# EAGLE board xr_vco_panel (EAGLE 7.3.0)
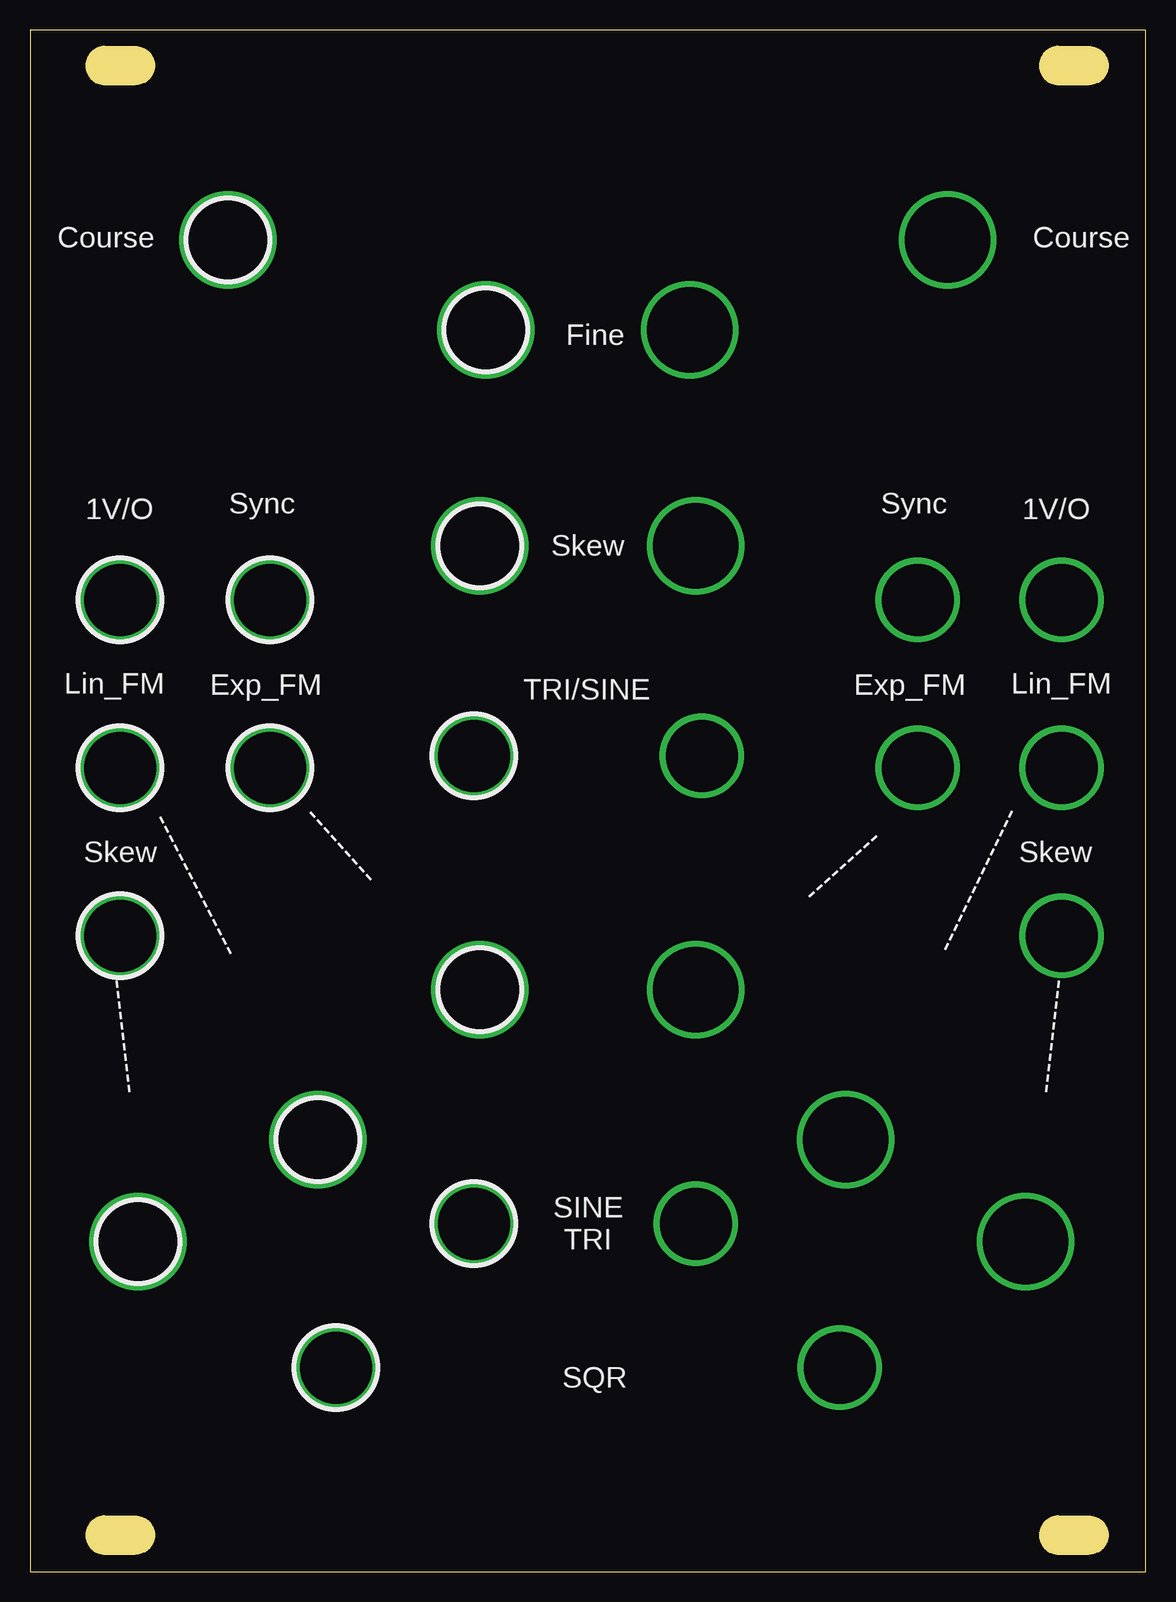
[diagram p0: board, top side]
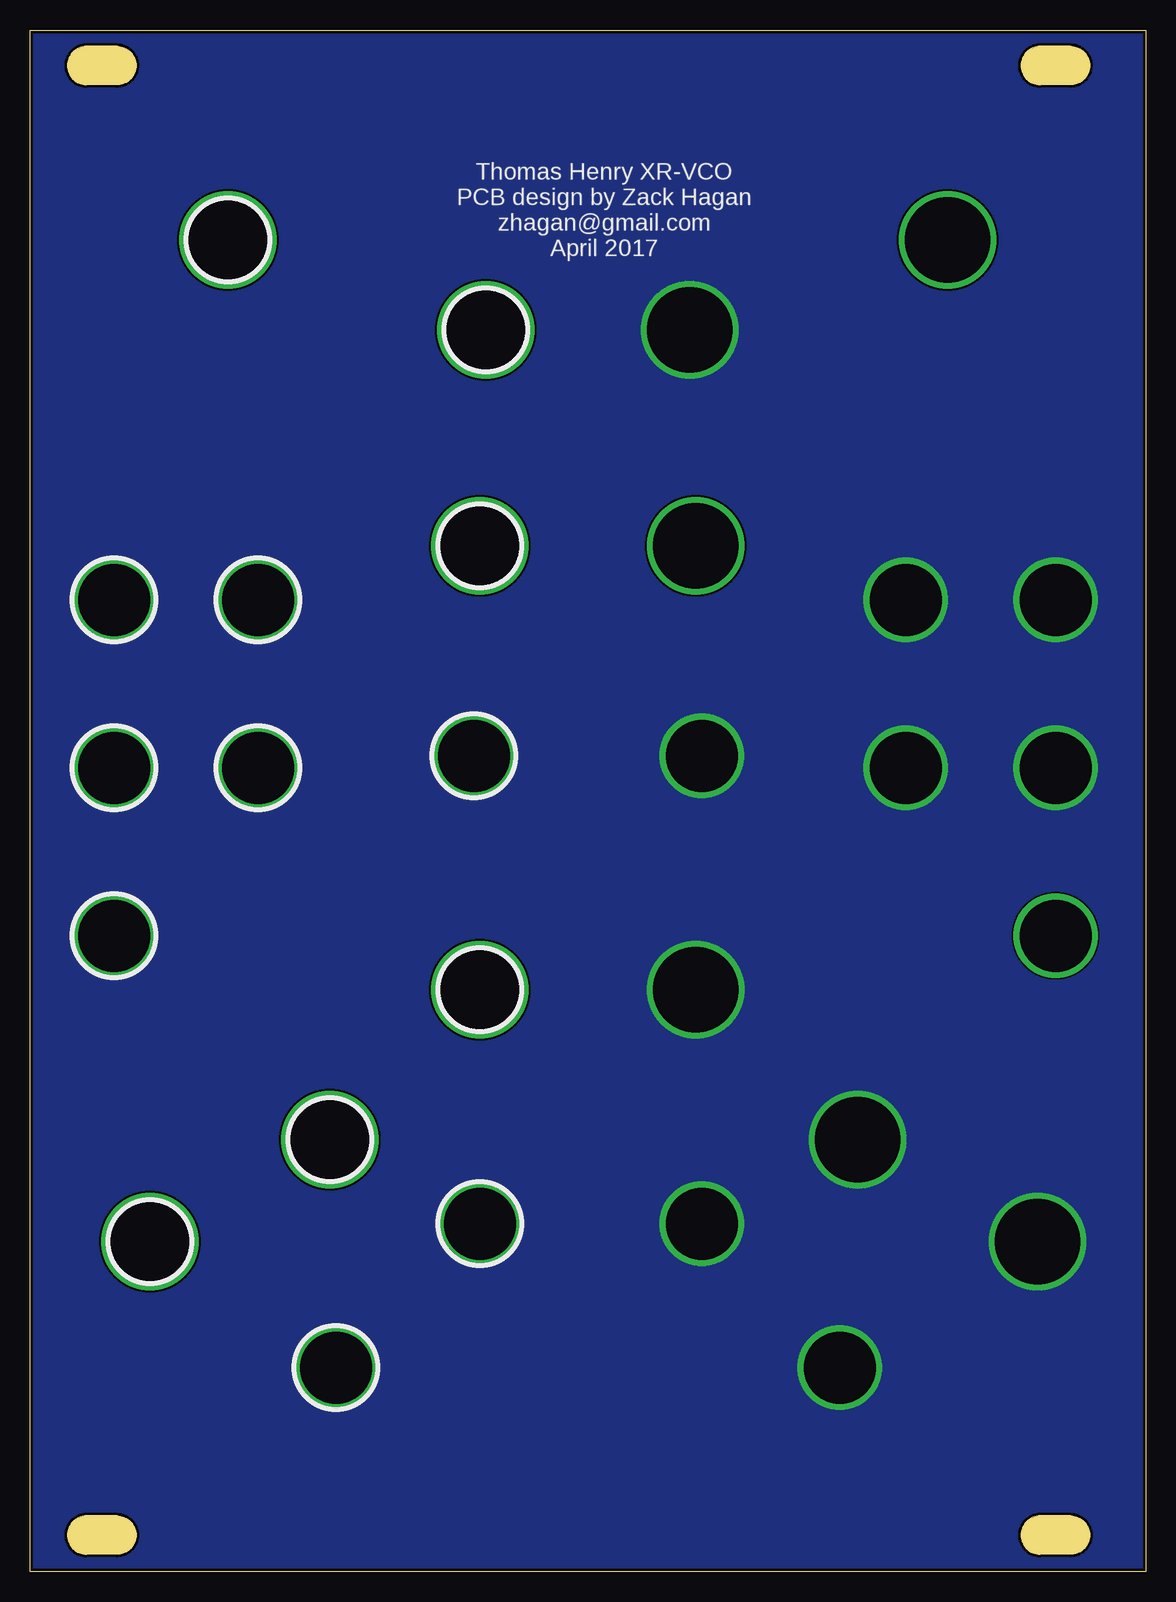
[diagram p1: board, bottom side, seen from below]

Size 93 x 128.5 mm. Coordinates in mm from the lower left corner, seen from the top.
Outline: 0,128.5 0,0 93,0 93,128.5 0,128.5
Copper layers (1*2*15*16): Top 0.035mm / dielectric 0.2mm / Route2 0.0175mm / dielectric 1.1mm / Route15 0.0175mm / dielectric 0.2mm / Bottom 0.035mm
Design rules "SeeedStudio_DRU_no_angle_20130527": minimum track width 6mil, minimum drill 12mil, track to track 6mil, track to pad 6mil, pad to pad 6mil, via to via 6mil, smd to smd 0mil, copper to edge 10mil, drill to drill 10mil, minimum pad ring 6mil, minimum via ring 6mil, stop-mask expansion 2mil, vias tented up to drill 25mil, thermal gap 10mil
Net classes: 1 power: width 0.406 mm; 2 ground: width 0.305 mm

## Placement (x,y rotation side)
U$1  [SLOT_HOLE]  87.02,125.53 0 top
U$2  [SLOT_HOLE]  87.02,3.04 0 top
U$3  [SLOT_HOLE]  7.52,125.53 0 top
U$4  [SLOT_HOLE]  7.52,3.04 0 top

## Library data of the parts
U$1-U$4 = MusicThingModular

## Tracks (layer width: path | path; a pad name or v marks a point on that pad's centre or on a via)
GND  (via drill 6, 7.1)
  other vias: 37,29 25.5,17 20,67 7.5,81 20,81 7.5,67 38,103.5 37,68 9,27.5 37.5,48.5 24,36 37.5,48.5
  pour Bottom: 95.56,130.31 96.1,-4.95 -2.86,-4.95 -5.4,130.31
GND1  (via drill 6)
  other vias: 7.5,53
GND2  (via drill 7.1)
  other vias: 16.5,111
GND3  (via drill 7.1)
  other vias: 37.5,85.5
GND4  (via drill 6, 7.1)
  other vias: 55.5,29 67.5,17 74,67 86,81 74,81 86,67 55,103.5 56,68 83,27.5 55.5,48.5 68,36 55.5,48.5
GND5  (via drill 6)
  other vias: 86,53
GND6  (via drill 7.1)
  other vias: 76.5,111
GND7  (via drill 7.1)
  other vias: 55.5,85.5

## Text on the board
tNames: Course | Course | Fine | 1V/O | Sync | Sync | 1V/O | Skew | Lin_FM | Exp_FM | TRI/SINE | Exp_FM | Lin_FM | --------------- | --------- | --------------- | --------- | Skew | Skew | ----------- | ----------- | SINE / TRI | SQR
bNames: Thomas Henry XR-VCO / PCB design by Zack Hagan / zhagan@gmail.com / April 2017
tStop: Dual XR-VCO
